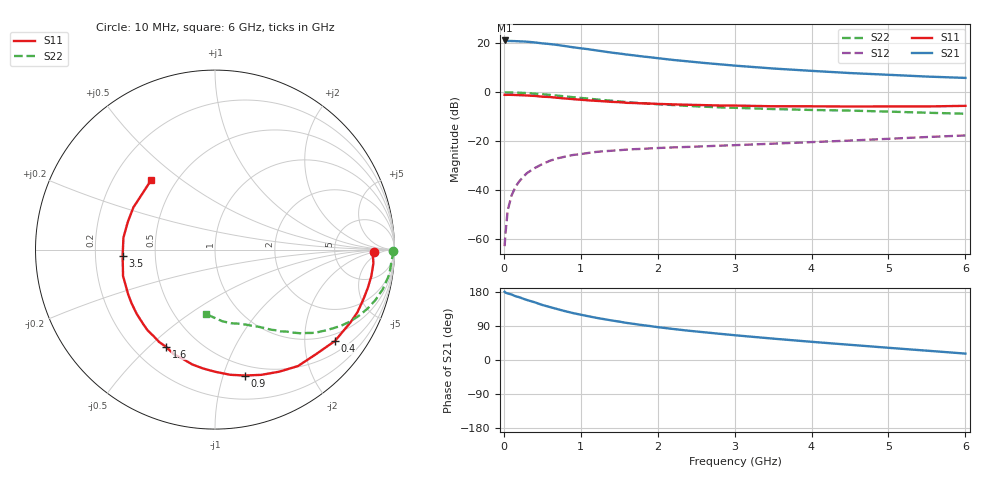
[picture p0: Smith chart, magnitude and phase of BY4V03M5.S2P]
! SIEMENS Small Signal Semiconductors
! BFY420
! Si NPN RF SIEGET Grounded Emitter Transistor in MICRO-X
! VCE = 4 V  IC = 3.5 mA
! Common Emitter S-Parameters:  October  1996
# GHz  S  MA  R  50
!  f  S11  S21  S12  S22
! GHz  MAG  ANG  MAG  ANG  MAG  ANG  MAG  ANG
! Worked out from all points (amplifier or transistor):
!   36 points, 10 MHz to 6 GHz, reference 50 ohm
!   highest |S21| = 21.2 dB at 10 MHz (marker M1)
!   |S21| within 3 dB of that: start of sweep to 948.8 MHz
!   unconditionally stable (mu >= 1): 3.451 GHz to end of sweep
!   at 250 MHz: K = 0.12, MSG = 27.8 dB, |S12| = -34.8 dB
!   at 1.4 GHz: K = 0.42, MSG = 20.1 dB, |S12| = -24.0 dB
!   at 6 GHz: K = 1.17, MAG = 9.3 dB, |S12| = -17.7 dB
!   S11 on the Smith chart (normalised r, x): 10 MHz: 16, -2; 400 MHz: 0.80, -2.76; 900 MHz: 0.40, -1.18; 1.6 GHz: 0.33, -0.57; 3.5 GHz: 0.32, -0.03; 6 GHz: 0.36, +0.39
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0.01  0.8858 -1.0  11.51 180.0  0.0007 31.1  0.9914 -0.3
0.02  0.88 -2.0  11.46 177.9  0.0012 61.5  0.9928 -0.9
0.05  0.8858 -4.9  11.24 175.6  0.0038 78.4  0.9898 -2.2
0.1  0.8835 -9.6  11.21 173.0  0.0076 81.4  0.9843 -4.5
0.15  0.8776 -14.2  11.15 168.4  0.0114 76.0  0.9818 -6.8
0.2  0.8714 -19.0  11.04 165.7  0.0149 78.0  0.9774 -8.9
0.25  0.8669 -23.8  10.98 161.9  0.0183 74.3  0.9682 -11.2
0.4  0.84 -37.3  10.5 152.4  0.0278 68.9  0.9367 -17.5
0.5  0.8101 -46.0  10.04 145.2  0.0337 64.7  0.9109 -21.2
0.6  0.7967 -54.5  9.709 139.7  0.0395 61.0  0.8816 -24.8
0.7  0.7688 -62.2  9.291 134.1  0.0443 57.6  0.852 -28.1
0.9  0.7212 -76.6  8.341 123.8  0.0518 51.0  0.7914 -33.6
1.1  0.6811 -89.8  7.607 115.4  0.057 46.6  0.7387 -38.4
1.3  0.6524 -101.2  6.843 107.9  0.0618 42.9  0.6902 -42.3
1.6  0.6061 -116.8  5.916 97.8  0.0667 38.4  0.6283 -47.3
2  0.5764 -133.9  4.99 86.7  0.0719 34.9  0.5675 -52.5
2.2  0.5642 -140.7  4.592 81.9  0.074 33.6  0.5458 -54.9
2.8  0.5354 -158.9  3.744 69.3  0.0802 31.5  0.4898 -61.1
3.5  0.5156 -176.3  3.063 56.4  0.0883 30.3  0.4524 -67.5
4.5  0.5097 162.3  2.473 40.1  0.1022 28.3  0.4202 -77.6
5.5  0.5112 141.9  2.094 24.6  0.1208 25.2  0.38 -90.4
6  0.526 132.6  1.966 16.9  0.1301 22.9  0.3626 -98.0
